| IBIS file stm32f413_f423_ufqfpn48.ibs
[IBIS ver] 4.2
[File name] stm32f413_f423_ufqfpn48.ibs
[File Rev] 1.2
[Date]  18-05-2020
[Source] Data Created at STMicroelectronics
[Notes]  File originated from ELDO simulations. rev 1.1: removal of the rising/falling waveform I2C
[Disclaimer]  This information is for modeling purpose only and is
   not guaranted. The information is subject to change without
   notice.
[Copyright] Copyright 2020 STMicroelectronics Inc.
|   Component stm32f413_f423_ufqfpn48
[Component] stm32f413_f423_ufqfpn48
[Manufacturer] STMicroelectronics
[Package]
| variable   typ   min   max
R_pkg   0.0   0.0   0.0
L_pkg   0.0H   0.0H   0.0H
C_pkg   0.0F   0.0F   0.0F
[Pin]  signal_name   model_name   R_pin   L_pin   C_pin
0 VSS_17  GND
1 VBAT POWER 0.053 3.42534E-09 90.4E-15
2 PC13-ANTI_TAMP io8p_arwsudq_ft_v33 48.4E-3 2.9E-9 64.4E-15
3 PC14-OSC32_IN io8p_arwsudq_ft 44.7E-3 2.5E-9 43.7E-15
4 PC15-OSC32_OUT io8p_arsudq_ft 41.9E-3 2.2E-9 28.1E-15
5 PH0-OSC_IN io8p_arsudq_ft 40.1E-3 2.0E-9 17.7E-15
6 PH1-OSC_OUT io8p_arsudq_ft 0.03913 1.89021E-09 12.5E-15
7 NRST ioreset_ft_v33 0.03913 1.89021E-09 12.5E-15
8 VSSA GND 40.1E-3 2.0E-9 17.8E-15
9 VDDA POWER 41.9E-3 2.2E-9 28.2E-15
10 PA0-WKUP io8p_arwsudq_ft_v33 44.7E-3 2.5E-9 43.8E-15
11 PA1 io8p_arwsudq_ft 48.4E-3 2.9E-9 64.6E-15
12 PA2 io8p_arwsudq_ft 0.053 3.42534E-09 90.4E-15
13 PA3 io8p_arwsudq_ft 0.053 3.4E-9 90.4E-15
14 PA4 io8p_ar3wsudq_ft 48.4E-3 2.9E-9 64.4E-15
15 PA5 io8p_ar3wsudq_ft 44.7E-3 2.5E-9 43.7E-15
16 PA6 io8p_ar3wsudq_ft 41.9E-3 2.2E-9 28.1E-15
17 PA7 io8p_arwsudq_ft 40.1E-3 2.0E-9 17.7E-15
18 PB0 io8p_ar3wsudq_ft 0.03913 1.9E-9 12.5E-15
19 PB1 io8p_ar3wsudq_ft 0.03913 1.9E-9 12.5E-15
20 PB2 io8p_arwsudq_ft 40.1E-3 2.0E-9 17.8E-15
21 PB10 io8p_arsudq_i2c_ft 41.9E-3 2.2E-9 28.2E-15
22 VCAP1_0 POWER 44.7E-3 2.5E-9 43.8E-15
23 VSS_1_1 GND 48.4E-3 2.9E-9 64.6E-15
24 VDD_1_0 POWER 0.053 3.4E-9 90.4E-15
25 PB12 io8p_arsudq_ft 0.053 3.4E-9 90.4E-15
26 PB13 io8p_arsudq_ft 48.4E-3 2.9E-9 64.4E-15
27 PB14 io8p_arsudq_i2c_ft 44.7E-3 2.5E-9 43.7E-15
28 PB15 io8p_arsudq_i2c_ft 41.9E-3 2.2E-9 28.1E-15
29 PA8 io8p_arsudq_i2cin_ft 40.1E-3 2.0E-9 17.7E-15
30 PA9 io8usb_vbus_otg_ft 0.03913 1.9E-9 12.5E-15
31 PA10 io8usb_id_otg_ft 0.03913 1.9E-9 12.5E-15
32 PA11 io8usb_lsfs_otg_ft 40.1E-3 2.0E-9 17.8E-15
33 PA12 io8usb_lsfs_otg_ft 41.9E-3 2.2E-9 28.2E-15
34 PA13 io8p_arsudq_ft 44.7E-3 2.5E-9 43.8E-15
35 VSS_2_0 GND 48.4E-3 2.9E-9 64.6E-15
36 VDD_SA_2 POWER 0.053 3.4E-9 90.4E-15
37 PA14 io8p_arsudq_ft 0.053 3.4E-9 90.4E-15
38 PA15 io8p_arsudq_ft 48.4E-3 2.9E-9 64.4E-15
39 PB3 io8p_arsudq_i2c_ft 44.7E-3 2.5E-9 43.7E-15
40 PB4 io8p_arsudq_i2cin_ft 41.9E-3 2.2E-9 28.1E-15
41 PB5 io8p_ar3wsudq_ft 40.1E-3 2.0E-9 17.7E-15
42 PB6 io8p_arsudq_i2cin_ft 0.03913 1.9E-9 12.5E-15
43 PB7 io8p_arsudq_i2cin_ft 0.03913 1.9E-9 12.5E-15
44 BOOT0 vpp_test_hv 40.1E-3 2.0E-9 17.8E-15
45 PB8 io8p_arsudq_i2cin_ft 41.9E-3 2.2E-9 28.2E-15
46 PB9 io8p_arsudq_i2cin_ft 44.7E-3 2.5E-9 43.8E-15
47 VSS_3 GND 48.4E-3 2.9E-9 64.6E-15
48 VDD_SA_3 POWER 0.053 3.4E-9 90.4E-15
[Model Selector] io8p_ar3wsudq_ft
io8p00_ar3wsudq_ft_pd_lv  "SPEED00 1P8V, PD=40kOhm"
io8p00_ar3wsudq_ft_pu_lv  "SPEED00 1P8V, PU=40kOhm"
io8p00_ar3wsudq_ft_lv  "SPEED00 1P8V"
io8p01_ar3wsudq_ft_pd_lv  "SPEED01 1P8V, PD=40kOhm"
io8p01_ar3wsudq_ft_pu_lv  "SPEED01 1P8V, PU=40kOhm"
io8p01_ar3wsudq_ft_lv  "SPEED01 1P8V"
io8p10_ar3wsudq_ft_pd_lv  "SPEED10 1P8V, PD=40kOhm"
io8p10_ar3wsudq_ft_pu_lv  "SPEED10 1P8V, PU=40kOhm"
io8p10_ar3wsudq_ft_lv  "SPEED10 1P8V"
io8p11_ar3wsudq_ft_pd_lv  "SPEED11 1P8V, PD=40kOhm"
io8p11_ar3wsudq_ft_pu_lv  "SPEED11 1P8V, PU=40kOhm"
io8p11_ar3wsudq_ft_lv  "SPEED11 1P8V"
io8p00_ar3wsudq_ft_pd  "SPEED00, PD=40kOhm"
io8p00_ar3wsudq_ft_pu  "SPEED00, PU=40kOhm"
io8p00_ar3wsudq_ft  "SPEED00"
io8p01_ar3wsudq_ft_pd  "SPEED01, PD=40kOhm"
io8p01_ar3wsudq_ft_pu  "SPEED01, PU=40kOhm"
io8p01_ar3wsudq_ft  "SPEED01"
io8p10_ar3wsudq_ft_pd  "SPEED10, PD=40kOhm"
io8p10_ar3wsudq_ft_pu  "SPEED10, PU=40kOhm"
io8p10_ar3wsudq_ft  "SPEED10"
io8p11_ar3wsudq_ft_pd  "SPEED11, PD=40kOhm"
io8p11_ar3wsudq_ft_pu  "SPEED11, PU=40kOhm"
io8p11_ar3wsudq_ft  "SPEED11"
[Model Selector] io8p_arsudq_ft
io8p00_arsudq_ft_pd_lv  "SPEED00 1P8V, PD=40kOhm"
io8p00_arsudq_ft_pu_lv  "SPEED00 1P8V, PU=40kOhm"
io8p00_arsudq_ft_lv  "SPEED00 1P8V"
io8p01_arsudq_ft_pd_lv  "SPEED01 1P8V, PD=40kOhm"
io8p01_arsudq_ft_pu_lv  "SPEED01 1P8V, PU=40kOhm"
io8p01_arsudq_ft_lv  "SPEED01 1P8V"
io8p10_arsudq_ft_pd_lv  "SPEED10 1P8V, PD=40kOhm"
io8p10_arsudq_ft_pu_lv  "SPEED10 1P8V, PU=40kOhm"
io8p10_arsudq_ft_lv  "SPEED10 1P8V"
io8p11_arsudq_ft_pd_lv  "SPEED11 1P8V, PD=40kOhm"
io8p11_arsudq_ft_pu_lv  "SPEED11 1P8V, PU=40kOhm"
io8p11_arsudq_ft_lv  "SPEED11 1P8V"
io8p00_arsudq_ft_pd  "SPEED00, PD=40kOhm"
io8p00_arsudq_ft_pu  "SPEED00, PU=40kOhm"
io8p00_arsudq_ft  "SPEED00"
io8p01_arsudq_ft_pd  "SPEED01, PD=40kOhm"
io8p01_arsudq_ft_pu  "SPEED01, PU=40kOhm"
io8p01_arsudq_ft  "SPEED01"
io8p10_arsudq_ft_pd  "SPEED10, PD=40kOhm"
io8p10_arsudq_ft_pu  "SPEED10, PU=40kOhm"
io8p10_arsudq_ft  "SPEED10"
io8p11_arsudq_ft_pd  "SPEED11, PD=40kOhm"
io8p11_arsudq_ft_pu  "SPEED11, PU=40kOhm"
io8p11_arsudq_ft  "SPEED11"
[Model Selector] io8p_arsudq_i2c_ft
io8prog_1v8_i2c_pd  "5V Tol GPIO 1.8V range i2c functionality with pull down"
io8prog_1v8_i2c_pu  "5V Tol GPIO 1.8V range i2c functionality with pull up"
io8prog_1v8_i2c  "5V Tol GPIO 1.8V range i2c functionality"
io8prog_3v3_i2c_pd  "5V Tol GPIO 3.3V range i2c functionality with pull down"
io8prog_3v3_i2c_pu  "5V Tol GPIO 3.3V range i2c functionality with pull up"
io8prog_3v3_i2c  "5V Tol GPIO 3.3V range i2c functionality"
io8prog_1v8_pd_00  "5V Tol GPIO 1.8V range with pd speed 00"
io8prog_1v8_pu_00  "5V Tol GPIO 1.8V range with pu speed 00"
io8prog_1v8_00  "5V Tol GPIO 1.8V range speed 00"
io8prog_3v3_pd_00  "5V Tol GPIO 3.3V range with pd speed 00"
io8prog_3v3_pu_00  "5V Tol GPIO 3.3V range with pu speed 00"
io8prog_3v3_00  "5V Tol GPIO 3.3V range speed 00"
io8prog_1v8_pd_01  "5V Tol GPIO 1.8V range with pd speed 01"
io8prog_1v8_pu_01  "5V Tol GPIO 1.8V range with pu speed 01"
io8prog_1v8_01  "5V Tol GPIO 1.8V range speed 01"
io8prog_3v3_pd_01  "5V Tol GPIO 3.3V range with pd speed 01"
io8prog_3v3_pu_01  "5V Tol GPIO 3.3V range with pu speed 01"
io8prog_3v3_01  "5V Tol GPIO 3.3V range speed 01"
io8prog_1v8_pd_10  "5V Tol GPIO 1.8V range with pd speed 10"
io8prog_1v8_pu_10  "5V Tol GPIO 1.8V range with pu speed 10"
io8prog_1v8_10  "5V Tol GPIO 1.8V range speed 10"
io8prog_3v3_pd_10  "5V Tol GPIO 3.3V range with pd speed 10"
io8prog_3v3_pu_10  "5V Tol GPIO 3.3V range with pu speed 10"
io8prog_3v3_10  "5V Tol GPIO 3.3V range speed 10"
io8prog_1v8_pd_11  "5V Tol GPIO 1.8V range with pd speed 11"
io8prog_1v8_pu_11  "5V Tol GPIO 1.8V range with pu speed 11"
io8prog_1v8_11  "5V Tol GPIO 1.8V range speed 11"
io8prog_3v3_pd_11  "5V Tol GPIO 3.3V range with pd speed 11"
io8prog_3v3_pu_11  "5V Tol GPIO 3.3V range with pu speed 11"
io8prog_3v3_11  "5V Tol GPIO 3.3V range speed 11"
[Model Selector] io8p_arsudq_i2cin_ft
io8p00_arsudq_i2cin_ft_pd_lv  "SPEED00 1P8V, PD=40kOhm"
io8p00_arsudq_i2cin_ft_pu_lv  "SPEED00 1P8V, PU=40kOhm"
io8p00_arsudq_i2cin_ft_lv  "SPEED00 1P8V"
io8p01_arsudq_i2cin_ft_pd_lv  "SPEED01 1P8V, PD=40kOhm"
io8p01_arsudq_i2cin_ft_pu_lv  "SPEED01 1P8V, PU=40kOhm"
io8p01_arsudq_i2cin_ft_lv  "SPEED01 1P8V"
io8p10_arsudq_i2cin_ft_pd_lv  "SPEED10 1P8V, PD=40kOhm"
io8p10_arsudq_i2cin_ft_pu_lv  "SPEED10 1P8V, PU=40kOhm"
io8p10_arsudq_i2cin_ft_lv  "SPEED10 1P8V"
io8p11_arsudq_i2cin_ft_pd_lv  "SPEED11 1P8V, PD=40kOhm"
io8p11_arsudq_i2cin_ft_pu_lv  "SPEED11 1P8V, PU=40kOhm"
io8p11_arsudq_i2cin_ft_lv  "SPEED11 1P8V"
io8p00_arsudq_i2cin_ft_pd  "SPEED00, PD=40kOhm"
io8p00_arsudq_i2cin_ft_pu  "SPEED00, PU=40kOhm"
io8p00_arsudq_i2cin_ft  "SPEED00"
io8p01_arsudq_i2cin_ft_pd  "SPEED01, PD=40kOhm"
io8p01_arsudq_i2cin_ft_pu  "SPEED01, PU=40kOhm"
io8p01_arsudq_i2cin_ft  "SPEED01"
io8p10_arsudq_i2cin_ft_pd  "SPEED10, PD=40kOhm"
io8p10_arsudq_i2cin_ft_pu  "SPEED10, PU=40kOhm"
io8p10_arsudq_i2cin_ft  "SPEED10"
io8p11_arsudq_i2cin_ft_pd  "SPEED11, PD=40kOhm"
io8p11_arsudq_i2cin_ft_pu  "SPEED11, PU=40kOhm"
io8p11_arsudq_i2cin_ft  "SPEED11"
[Model Selector] io8p_arwsudq_ft
io8p00_arwsudq_ft_pd_lv  "SPEED00 1P8V, PD=40kOhm"
io8p00_arwsudq_ft_pu_lv  "SPEED00 1P8V, PU=40kOhm"
io8p00_arwsudq_ft_lv  "SPEED00 1P8V"
io8p01_arwsudq_ft_pd_lv  "SPEED01 1P8V, PD=40kOhm"
io8p01_arwsudq_ft_pu_lv  "SPEED01 1P8V, PU=40kOhm"
io8p01_arwsudq_ft_lv  "SPEED01 1P8V"
io8p10_arwsudq_ft_pd_lv  "SPEED10 1P8V, PD=40kOhm"
io8p10_arwsudq_ft_pu_lv  "SPEED10 1P8V, PU=40kOhm"
io8p10_arwsudq_ft_lv  "SPEED10 1P8V"
io8p11_arwsudq_ft_pd_lv  "SPEED11 1P8V, PD=40kOhm"
io8p11_arwsudq_ft_pu_lv  "SPEED11 1P8V, PU=40kOhm"
io8p11_arwsudq_ft_lv  "SPEED11 1P8V"
io8p00_arwsudq_ft_pd  "SPEED00, PD=40kOhm"
io8p00_arwsudq_ft_pu  "SPEED00, PU=40kOhm"
io8p00_arwsudq_ft  "SPEED00"
io8p01_arwsudq_ft_pd  "SPEED01, PD=40kOhm"
io8p01_arwsudq_ft_pu  "SPEED01, PU=40kOhm"
io8p01_arwsudq_ft  "SPEED01"
io8p10_arwsudq_ft_pd  "SPEED10, PD=40kOhm"
io8p10_arwsudq_ft_pu  "SPEED10, PU=40kOhm"
io8p10_arwsudq_ft  "SPEED10"
io8p11_arwsudq_ft_pd  "SPEED11, PD=40kOhm"
io8p11_arwsudq_ft_pu  "SPEED11, PU=40kOhm"
io8p11_arwsudq_ft  "SPEED11"
[Model Selector] io8p_arwsudq_ft_v33
io8p00_arwsudq_ft_v33_pd_lv  "SPEED00 1P8V, PD=40kOhm"
io8p00_arwsudq_ft_v33_pu_lv  "SPEED00 1P8V, PU=40kOhm"
io8p00_arwsudq_ft_v33_lv  "SPEED00 1P8V"
io8p01_arwsudq_ft_v33_pd_lv  "SPEED01 1P8V, PD=40kOhm"
io8p01_arwsudq_ft_v33_pu_lv  "SPEED01 1P8V, PU=40kOhm"
io8p01_arwsudq_ft_v33_lv  "SPEED01 1P8V"
io8p10_arwsudq_ft_v33_pd_lv  "SPEED10 1P8V, PD=40kOhm"
io8p10_arwsudq_ft_v33_pu_lv  "SPEED10 1P8V, PU=40kOhm"
io8p10_arwsudq_ft_v33_lv  "SPEED10 1P8V"
io8p11_arwsudq_ft_v33_pd_lv  "SPEED11 1P8V, PD=40kOhm"
io8p11_arwsudq_ft_v33_pu_lv  "SPEED11 1P8V, PU=40kOhm"
io8p11_arwsudq_ft_v33_lv  "SPEED11 1P8V"
io8p00_arwsudq_ft_v33_pd  "SPEED00, PD=40kOhm"
io8p00_arwsudq_ft_v33_pu  "SPEED00, PU=40kOhm"
io8p00_arwsudq_ft_v33  "SPEED00"
io8p01_arwsudq_ft_v33_pd  "SPEED01, PD=40kOhm"
io8p01_arwsudq_ft_v33_pu  "SPEED01, PU=40kOhm"
io8p01_arwsudq_ft_v33  "SPEED01"
io8p10_arwsudq_ft_v33_pd  "SPEED10, PD=40kOhm"
io8p10_arwsudq_ft_v33_pu  "SPEED10, PU=40kOhm"
io8p10_arwsudq_ft_v33  "SPEED10"
io8p11_arwsudq_ft_v33_pd  "SPEED11, PD=40kOhm"
io8p11_arwsudq_ft_v33_pu  "SPEED11, PU=40kOhm"
io8p11_arwsudq_ft_v33  "SPEED11"
[Model Selector] io8usb_id_otg_ft
io8p00_id_otg_ft_pd_lv  "SPEED00 1P8V, PD=14kOhm"
io8p00_id_otg_ft_pu_lv  "SPEED00 1P8V, PU=14kOhm"
io8p00_id_otg_ft_lv  "SPEED00 1P8V"
io8p01_id_otg_ft_pd_lv  "SPEED01 1P8V, PD=14kOhm"
io8p01_id_otg_ft_pu_lv  "SPEED01 1P8V, PU=14kOhm"
io8p01_id_otg_ft_lv  "SPEED01 1P8V"
io8p10_id_otg_ft_pd_lv  "SPEED10 1P8V, PD=14kOhm"
io8p10_id_otg_ft_pu_lv  "SPEED10 1P8V, PU=14kOhm"
io8p10_id_otg_ft_lv  "SPEED10 1P8V"
io8p11_id_otg_ft_pd_lv  "SPEED11 1P8V, PD=14kOhm"
io8p11_id_otg_ft_pu_lv  "SPEED11 1P8V, PU=14kOhm"
io8p11_id_otg_ft_lv  "SPEED11 1P8V"
io8p00_id_otg_ft_pd  "SPEED00, PD=14kOhm"
io8p00_id_otg_ft_pu  "SPEED00, PU=14kOhm"
io8p00_id_otg_ft  "SPEED00"
io8p01_id_otg_ft_pd  "SPEED01, PD=14kOhm"
io8p01_id_otg_ft_pu  "SPEED01, PU=14kOhm"
io8p01_id_otg_ft  "SPEED01"
io8p10_id_otg_ft_pd  "SPEED10, PD=14kOhm"
io8p10_id_otg_ft_pu  "SPEED10, PU=14kOhm"
io8p10_id_otg_ft  "SPEED10"
io8p11_id_otg_ft_pd  "SPEED11, PD=14kOhm"
io8p11_id_otg_ft_pu  "SPEED11, PU=14kOhm"
io8p11_id_otg_ft  "SPEED11"
[Model Selector] io8usb_lsfs_otg_ft
io8usb_ls_otg_ft_dpdn_pd  "LS USB DP/DN IO + PD=20kOhm"
io8usb_ls_otg_ft_dpdn_pupu2  "LS USB DP/DN IO + PU/PU2=2.2kOhm"
io8usb_ls_otg_ft_dpdn_pu2  "LS USB DP/DN IO + PU2=1.2kOhm"
io8usb_ls_otg_ft_dpdn_pu  "LS USB DP/DN IO + PU=1.2kOhm"
io8usb_ls_otg_ft_dpdn  "LS USB DP/DN IO"
io8usb_fs_otg_ft_dpdn_pd  "HS USB DP/DN IO + PD=20kOhm"
io8usb_fs_otg_ft_dpdn_pupu2  "HS USB DP/DN IO + PU/PU2=2.2kOhm"
io8usb_fs_otg_ft_dpdn_pu2  "HS USB DP/DN IO + PU2=1.2kOhm"
io8usb_fs_otg_ft_dpdn_pu  "HS USB DP/DN IO + PU=1.2kOhm"
io8usb_fs_otg_ft_dpdn  "HS USB DP/DN IO"
io8p00_lsfs_otg_ft_pd_lv  "SPEED00 1P8V, PD=40kOhm"
io8p00_lsfs_otg_ft_pu_lv  "SPEED00 1P8V, PU=40kOhm"
io8p00_lsfs_otg_ft_lv  "SPEED00 1P8V"
io8p01_lsfs_otg_ft_pd_lv  "SPEED01 1P8V, PD=40kOhm"
io8p01_lsfs_otg_ft_pu_lv  "SPEED01 1P8V, PU=40kOhm"
io8p01_lsfs_otg_ft_lv  "SPEED01 1P8V"
io8p10_lsfs_otg_ft_pd_lv  "SPEED10 1P8V, PD=40kOhm"
io8p10_lsfs_otg_ft_pu_lv  "SPEED10 1P8V, PU=40kOhm"
io8p10_lsfs_otg_ft_lv  "SPEED10 1P8V"
io8p11_lsfs_otg_ft_pd_lv  "SPEED11 1P8V, PD=40kOhm"
io8p11_lsfs_otg_ft_pu_lv  "SPEED11 1P8V, PU=40kOhm"
io8p11_lsfs_otg_ft_lv  "SPEED11 1P8V"
io8p00_lsfs_otg_ft_pd  "SPEED00, PD=40kOhm"
io8p00_lsfs_otg_ft_pu  "SPEED00, PU=40kOhm"
io8p00_lsfs_otg_ft  "SPEED00"
io8p01_lsfs_otg_ft_pd  "SPEED01, PD=40kOhm"
io8p01_lsfs_otg_ft_pu  "SPEED01, PU=40kOhm"
io8p01_lsfs_otg_ft  "SPEED01"
io8p10_lsfs_otg_ft_pd  "SPEED10, PD=40kOhm"
io8p10_lsfs_otg_ft_pu  "SPEED10, PU=40kOhm"
io8p10_lsfs_otg_ft  "SPEED10"
io8p11_lsfs_otg_ft_pd  "SPEED11, PD=40kOhm"
io8p11_lsfs_otg_ft_pu  "SPEED11, PU=40kOhm"
io8p11_lsfs_otg_ft  "SPEED11"
[Model Selector] io8usb_vbus_otg_ft
io8psenb_vbus_otg_ft  "VBUS PULSE, SENSE VB"
io8psenab_vbus_otg_ft  "VBUS PULSE, SENSE VA and VB"
io8psena_vbus_otg_ft  "VBUS PULSE, SENSE VA"
io8psen_vbus_otg_ft  "VBUS PULSE"
io8p00_vbus_otg_ft_pd_lv  "SPEED00 1P8V, PD=40kOhm"
io8p00_vbus_otg_ft_pu_lv  "SPEED00 1P8V, PU=40kOhm"
io8p00_vbus_otg_ft_lv  "SPEED00 1P8V"
io8p01_vbus_otg_ft_pd_lv  "SPEED01 1P8V, PD=40kOhm"
io8p01_vbus_otg_ft_pu_lv  "SPEED01 1P8V, PU=40kOhm"
io8p01_vbus_otg_ft_lv  "SPEED01 1P8V"
io8p10_vbus_otg_ft_pd_lv  "SPEED10 1P8V, PD=40kOhm"
io8p10_vbus_otg_ft_pu_lv  "SPEED10 1P8V, PU=40kOhm"
io8p10_vbus_otg_ft_lv  "SPEED10 1P8V"
io8p11_vbus_otg_ft_pd_lv  "SPEED11 1P8V, PD=40kOhm"
io8p11_vbus_otg_ft_pu_lv  "SPEED11 1P8V, PU=40kOhm"
io8p11_vbus_otg_ft_lv  "SPEED11 1P8V"
io8p00_vbus_otg_ft_pd  "SPEED00, PD=40kOhm"
io8p00_vbus_otg_ft_pu  "SPEED00, PU=40kOhm"
io8p00_vbus_otg_ft  "SPEED00"
io8p01_vbus_otg_ft_pd  "SPEED01, PD=40kOhm"
io8p01_vbus_otg_ft_pu  "SPEED01, PU=40kOhm"
io8p01_vbus_otg_ft  "SPEED01"
io8p10_vbus_otg_ft_pd  "SPEED10, PD=40kOhm"
io8p10_vbus_otg_ft_pu  "SPEED10, PU=40kOhm"
io8p10_vbus_otg_ft  "SPEED10"
io8p11_vbus_otg_ft_pd  "SPEED11, PD=40kOhm"
io8p11_vbus_otg_ft_pu  "SPEED11, PU=40kOhm"
io8p11_vbus_otg_ft  "SPEED11"
[Model Selector] ioreset_ft_v33
ioreset_ft_v33_pu_lv  "IORESET 1P8V + PU=40kOhm"
ioreset_ft_v33_nopu_lv  "IORESET 1P8V"
ioreset_ft_v33_pu  "IORESET + PU=40kOhm"
ioreset_ft_v33_nopu  "IORESET"
[Model Selector] vpp_test_hv
vpp_test_hv_2p4  "Input Buffer 1P8V"
vpp_test_hv_3p3  "Input Buffer"
| Models and submodels in the file (242): io8p00_ar3wsudq_ft_pd_lv (I/O), io8p00_ar3wsudq_ft_pu_lv (I/O), io8p00_ar3wsudq_ft_lv (I/O), io8p01_ar3wsudq_ft_pd_lv (I/O), io8p01_ar3wsudq_ft_pu_lv (I/O), io8p01_ar3wsudq_ft_lv (I/O), io8p10_ar3wsudq_ft_pd_lv (I/O), io8p10_ar3wsudq_ft_pu_lv (I/O), io8p10_ar3wsudq_ft_lv (I/O), io8p11_ar3wsudq_ft_pd_lv (I/O), io8p11_ar3wsudq_ft_pu_lv (I/O), io8p11_ar3wsudq_ft_lv (I/O), io8p00_ar3wsudq_ft_pd (I/O), io8p00_ar3wsudq_ft_pu (I/O), io8p00_ar3wsudq_ft (I/O), io8p01_ar3wsudq_ft_pd (I/O), io8p01_ar3wsudq_ft_pu (I/O), io8p01_ar3wsudq_ft (I/O), io8p10_ar3wsudq_ft_pd (I/O), io8p10_ar3wsudq_ft_pu (I/O), io8p10_ar3wsudq_ft (I/O), io8p11_ar3wsudq_ft_pd (I/O), io8p11_ar3wsudq_ft_pu (I/O), io8p11_ar3wsudq_ft (I/O), io8p00_arsudq_ft_pd_lv (I/O), io8p00_arsudq_ft_pu_lv (I/O), io8p00_arsudq_ft_lv (I/O), io8p01_arsudq_ft_pd_lv (I/O), io8p01_arsudq_ft_pu_lv (I/O), io8p01_arsudq_ft_lv (I/O), io8p10_arsudq_ft_pd_lv (I/O), io8p10_arsudq_ft_pu_lv (I/O), io8p10_arsudq_ft_lv (I/O), io8p11_arsudq_ft_pd_lv (I/O), io8p11_arsudq_ft_pu_lv (I/O), io8p11_arsudq_ft_lv (I/O), io8p00_arsudq_ft_pd (I/O), io8p00_arsudq_ft_pu (I/O), io8p00_arsudq_ft (I/O), io8p01_arsudq_ft_pd (I/O), io8p01_arsudq_ft_pu (I/O), io8p01_arsudq_ft (I/O), io8p10_arsudq_ft_pd (I/O), io8p10_arsudq_ft_pu (I/O), io8p10_arsudq_ft (I/O), io8p11_arsudq_ft_pd (I/O), io8p11_arsudq_ft_pu (I/O), io8p11_arsudq_ft (I/O), io8prog_1v8_i2c_pd (I/O), io8prog_1v8_i2c_pu (I/O), io8prog_1v8_i2c (I/O), io8prog_3v3_i2c_pd (I/O), io8prog_3v3_i2c_pu (I/O), io8prog_3v3_i2c (I/O), io8prog_1v8_pd_00 (I/O), io8prog_1v8_pu_00 (I/O), io8prog_1v8_00 (I/O), io8prog_3v3_pd_00 (I/O), io8prog_3v3_pu_00 (I/O), io8prog_3v3_00 (I/O), io8prog_1v8_pd_01 (I/O), io8prog_1v8_pu_01 (I/O), io8prog_1v8_01 (I/O), io8prog_3v3_pd_01 (I/O), io8prog_3v3_pu_01 (I/O), io8prog_3v3_01 (I/O), io8prog_1v8_pd_10 (I/O), io8prog_1v8_pu_10 (I/O), io8prog_1v8_10 (I/O), io8prog_3v3_pd_10 (I/O), io8prog_3v3_pu_10 (I/O), io8prog_3v3_10 (I/O), io8prog_1v8_pd_11 (I/O), io8prog_1v8_pu_11 (I/O), io8prog_1v8_11 (I/O), io8prog_3v3_pd_11 (I/O), io8prog_3v3_pu_11 (I/O), io8prog_3v3_11 (I/O), io8p00_arsudq_i2cin_ft_pd_lv (I/O), io8p00_arsudq_i2cin_ft_pu_lv (I/O)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
